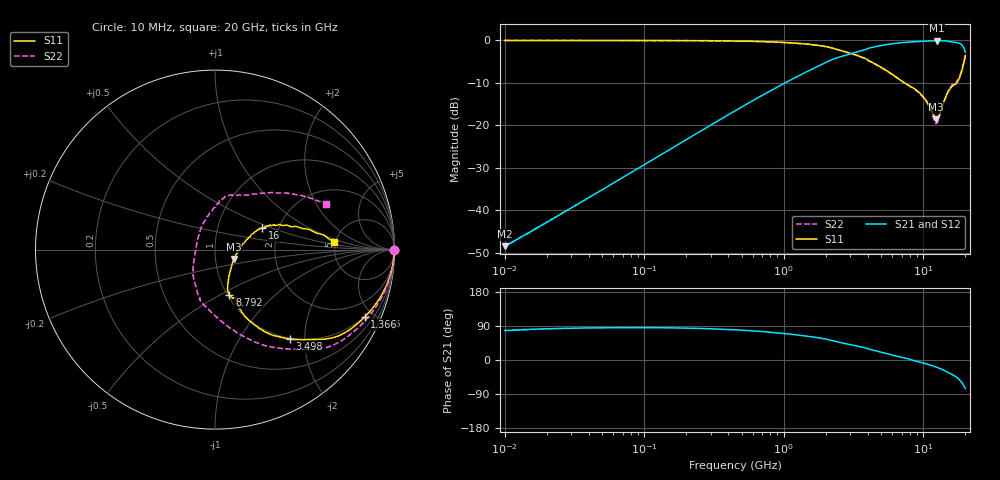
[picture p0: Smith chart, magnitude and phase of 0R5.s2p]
!Keysight Technologies,P5008B,MY61100088,A.16.20.02
!Date: Monday, October 30, 2023 15:52:23
!Correction: S11(C  2-Port  )
!S21(C  2-Port  )
!S12(C  2-Port  )
!S22(C  2-Port  )
!S2P File: Measurements: S11, S21, S12, S22:Log Frequency Sweep
# Hz S  dB  R 50
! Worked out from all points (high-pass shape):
!   1601 points, 10 MHz to 20 GHz, reference 50 ohm
!   highest |S21| = -0.03 dB at 12.5 GHz (marker M1); lowest = -48.4 dB at 10.05 MHz (marker M2)
!   |S21| within 3 dB of the highest: 3.099 GHz to end of sweep
!   lowest |S11| = -18.6 dB at 12.38 GHz (marker M3), VSWR 1.27, Z = 61.4 - j6.47 ohm
!   |S11| at or under -10 dB: 7.362 GHz to 17.27 GHz (9.912 GHz wide, 80.5 % of centre)
!   |S22| runs from -19.5 to 0.0 dB; largest |S21 - S12| = 0.0012
!   S11 on the Smith chart (normalised r, x): 10 MHz: open; 1.366 GHz: 0.97, -4.46; 3.498 GHz: 0.99, -1.69; 8.792 GHz: 1.02, -0.55; 16 GHz: 1.64, +0.43; 20 GHz: 4.83, +0.76
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1e7  -0.00 -0.2  -48.42 78.2  -48.44 78.9  -0.01 -0.2
1.004762e7  -0.00 -0.2  -48.43 77.8  -48.39 78.6  -0.01 -0.2
3.555162e7  -0.01 -0.7  -38.00 84.2  -38.02 84.2  -0.01 -0.8
1.263918e8  -0.02 -2.5  -27.27 85.1  -27.28 85.1  -0.03 -2.8
4.472136e8  -0.13 -8.6  -16.58 79.7  -16.58 79.7  -0.13 -9.7
8.3724e8  -0.35 -15.6  -11.50 72.8  -11.50 72.8  -0.36 -17.6
1.365695e9  -0.77 -24.2  -7.84 64.5  -7.84 64.5  -0.77 -27.5
1.589917e9  -0.98 -27.7  -6.76 61.3  -6.77 61.3  -0.98 -31.5
2.238313e9  -1.82 -37.5  -4.44 51.0  -4.44 51.0  -1.83 -42.9
3.498293e9  -3.75 -50.0  -2.51 35.4  -2.51 35.4  -3.77 -57.8
5.652411e9  -7.43 -64.9  -0.89 15.4  -0.90 15.4  -7.49 -82.2
7.552409e9  -10.27 -67.2  -0.43 4.1  -0.43 4.1  -10.30 -103.5
8.792373e9  -11.57 -72.2  -0.29 -2.7  -0.29 -2.6  -11.69 -111.9
1.043228e10  -14.09 -68.4  -0.15 -9.9  -0.15 -9.9  -14.23 -128.4
1.237806e10  -18.60 -26.3  -0.04 -18.6  -0.04 -18.5  -19.48 169.3
1.249622e10  -18.53 -21.2  -0.03 -19.2  -0.04 -19.1  -19.47 161.9
1.304209e10  -17.48 -0.7  -0.06 -21.9  -0.06 -21.9  -17.81 131.8
1.475668e10  -12.68 23.0  -0.17 -31.3  -0.18 -31.3  -12.67 91.3
1.599787e10  -10.80 24.8  -0.37 -37.8  -0.37 -37.8  -10.49 79.5
1.810106e10  -8.89 22.5  -0.65 -51.8  -0.65 -51.7  -8.53 55.7
1.898171e10  -6.82 16.3  -1.14 -61.0  -1.15 -60.9  -6.59 42.4
2e10  -3.56 3.8  -2.78 -75.5  -2.79 -75.5  -3.48 22.3
